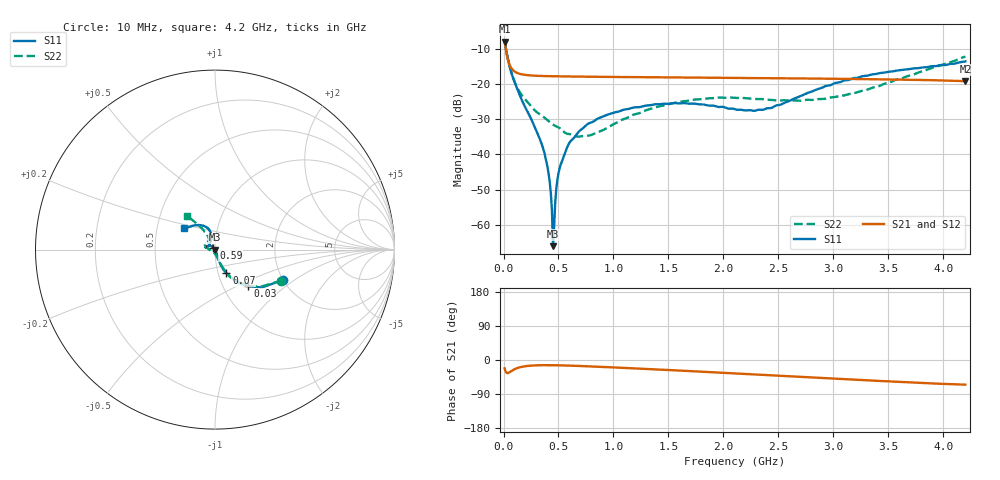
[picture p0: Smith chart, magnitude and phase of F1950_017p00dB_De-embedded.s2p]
! Integrated Device Technology
! Corporate Headquarters
! 6024 Silver Creek Valley Road
! San Jose, CA 95138  USA
! Phone:  1-408-284-8200
! Toll Free:  1-800-223-1366
! Webpage:  http://www.idt.com/
! Timing and RF Division
! 515 Groton Road, Suite 102
! Westford, MA 01886-6024
! Device:  F1950
! Description: 7-bit 0.25 dB Digital Step Attenuator
! Frequency:  150.0 -  4000.00 MHz
! Package:  4x4 mm Thin QFN Plastic Package: 24 pin
! Ports:  2 RF, 12 DC
!  Pin  1  = D0
!  Pin  2  = VDD
!  Pin  3  = Vmode
!  Pin  4  = GND
!  Pin  5  = RF1  =  Port 1
!  Pin  6  = GND
!  Pin  7  = GND
!  Pin  8  = GND
!  Pin  9  = GND
!  Pin 10  = GND
!  Pin 11  = GND
!  Pin 12  = GND
!  Pin 13  = GND
!  Pin 14  = RF2  =  Port 2
!  Pin 15  = GND
!  Pin 16  = LE
!  Pin 17  = CLK
!  Pin 18  = DATE
!  Pin 19  = D6
!  Pin 20  = D5
!  Pin 21  = D4
!  Pin 22  = D3
!  Pin 23  = D2
!  Pin 24  = D1
! State:  68
! Atten State:  17.00 dB
! Voltage:  +5.00 Volts
! Current:  Not Measured mA
! Data:  The device was measured on a the F195X evaluation board which has
!  individual transmission lines to the RF pins.  Data was collected
!  using a calibrated network analyzer.  The evaluation board was
!  de-embedded using a TRL calibration technique.
!  The reference plane is the edge of the package pin.
! Misc:  Board 2019
!  Action Tracker AT0250
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# GHz S dB R 50
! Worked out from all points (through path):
!   420 points, 10 MHz to 4.2 GHz, reference 50 ohm
!   highest |S21| = -7.96 dB at 10 MHz (marker M1); lowest = -19.2 dB at 4.2 GHz (marker M2)
!   group delay of S21, straight-line fit = 36.3 ps
!   lowest |S11| = -66.1 dB at 450 MHz (marker M3), VSWR 1.00, Z = 50 - j0.0492 ohm
!   |S11| at or under -10 dB: 22.87 MHz to end of sweep
!   |S22| runs from -35.0 to -7.8 dB; largest |S21 - S12| = 0.0002
!   S11 on the Smith chart (normalised r, x): 10 MHz: 2.00, -0.82; 30 MHz: 1.30, -0.57; 70 MHz: 1.10, -0.30; 590 MHz: 0.98, +0.02; 4.2 GHz: 0.69, +0.17
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0.01  -7.62 -24.0  -7.96 -22.2  -7.96 -22.2  -7.80 -25.1
0.03  -11.28 -48.0  -11.70 -34.3  -11.70 -34.3  -11.38 -48.2
0.07  -16.68 -64.1  -15.42 -29.4  -15.42 -29.4  -16.51 -63.5
0.16  -24.09 -70.3  -17.21 -18.4  -17.21 -18.4  -22.90 -71.3
0.36  -38.30 -63.4  -17.73 -13.7  -17.73 -13.7  -29.26 -79.4
0.41  -45.47 -66.0  -17.77 -13.7  -17.77 -13.7  -30.54 -80.9
0.44  -55.65 -74.8  -17.79 -13.8  -17.79 -13.8  -31.31 -84.4
0.45  -66.07 -97.9  -17.80 -13.8  -17.80 -13.8  -31.52 -85.8
0.47  -53.76 125.5  -17.81 -13.9  -17.81 -13.9  -31.87 -88.8
0.49  -47.15 125.5  -17.82 -14.0  -17.82 -14.0  -32.16 -91.0
0.51  -43.96 128.1  -17.83 -14.1  -17.83 -14.1  -32.51 -92.3
0.59  -37.22 130.3  -17.86 -14.7  -17.86 -14.8  -34.17 -105.4
0.71  -32.86 134.9  -17.90 -16.0  -17.90 -16.0  -34.84 -127.0
0.99  -28.27 145.8  -17.99 -19.4  -17.99 -19.4  -31.61 -171.0
1.41  -25.74 162.3  -18.10 -25.2  -18.10 -25.2  -26.38 167.0
1.73  -25.55 167.8  -18.18 -29.8  -18.18 -29.8  -24.46 158.3
2.11  -27.22 157.0  -18.27 -35.6  -18.27 -35.6  -23.94 149.1
2.43  -26.83 125.0  -18.35 -40.2  -18.35 -40.2  -24.50 139.4
2.81  -22.06 104.4  -18.45 -46.1  -18.44 -46.1  -24.52 124.6
3.19  -18.30 107.8  -18.57 -52.0  -18.57 -52.0  -22.59 117.8
3.51  -16.48 116.7  -18.70 -56.6  -18.70 -56.6  -19.59 118.8
4.2  -13.55 145.6  -19.19 -65.1  -19.18 -65.2  -12.20 129.5
